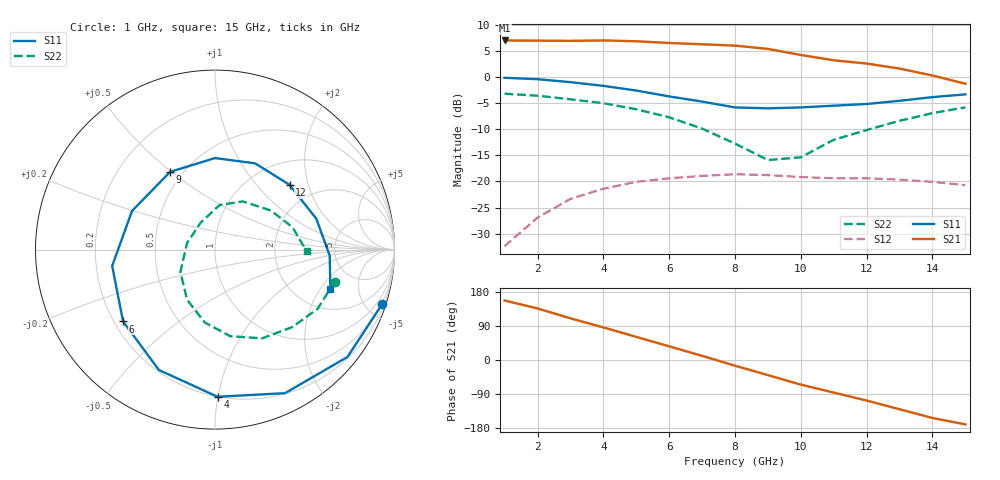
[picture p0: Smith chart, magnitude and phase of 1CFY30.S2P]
!CFY30 1æ GaAs FET in SOT143 package
!V DS = 3.5V, I D = 15mA, Z 0 = 50 Ohm
# GHZ S MA R 50
!f GHz  S11  S21  S12  S22
!  MAG  ANG  MAG  ANG  MAG  ANG  MAG  ANG
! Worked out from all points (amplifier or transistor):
!   15 points, 1 GHz to 15 GHz, reference 50 ohm
!   highest |S21| = 7.0 dB at 1 GHz (marker M1)
!   |S21| within 3 dB of that: start of sweep to 10.22 GHz
!   unconditionally stable (mu >= 1): 5.217 GHz to end of sweep
!   at 3 GHz: K = 0.61, MSG = 15.1 dB, |S12| = -23.3 dB
!   at 8 GHz: K = 1.57, MAG = 7.9 dB, |S12| = -18.6 dB
!   at 15 GHz: K = 2.49, MAG = 2.9 dB, |S12| = -20.7 dB
!   S11 on the Smith chart (normalised r, x): 1 GHz: 0.41, -6.29; 4 GHz: 0.20, -1.00; 6 GHz: 0.24, -0.33; 9 GHz: 0.43, +0.49; 12 GHz: 1.48, +1.53; 15 GHz: 3.05, -2.51
1  0.98 -18.0  2.23 157.0  0.024 74.0  0.69 -15.0
2  0.95 -39.0  2.22 136.0  0.045 57.0  0.66 -30.0
3  0.89 -64.0  2.21 110.0  0.068 40.0  0.61 -45.0
4  0.82 -89.0  2.23 86.0  0.085 23.0  0.56 -62.0
5  0.74 -115.0  2.19 61.0  0.099 7.0  0.49 -80.0
6  0.65 -142.0  2.11 36.0  0.107 -10.0  0.41 -98.0
7  0.58 -171.0  2.05 11.0  0.113 -26.0  0.32 -119.0
8  0.51 155.0  1.99 -15.0  0.117 -41.0  0.23 -147.0
9  0.5 120.0  1.85 -40.0  0.115 -56.0  0.16 167.0
10  0.51 90.0  1.62 -65.0  0.11 -69.0  0.17 118.0
11  0.53 65.0  1.44 -86.0  0.107 -80.0  0.25 84.0
12  0.55 41.0  1.34 -107.0  0.107 -92.0  0.31 60.0
13  0.59 17.0  1.2 -130.0  0.104 -105.0  0.38 35.0
14  0.64 -3.0  1.03 -153.0  0.099 -118.0  0.45 16.0
15  0.68 -19.0  0.86 -170.0  0.092 -131.0  0.51 -1.0
